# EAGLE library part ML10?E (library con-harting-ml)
HARTING
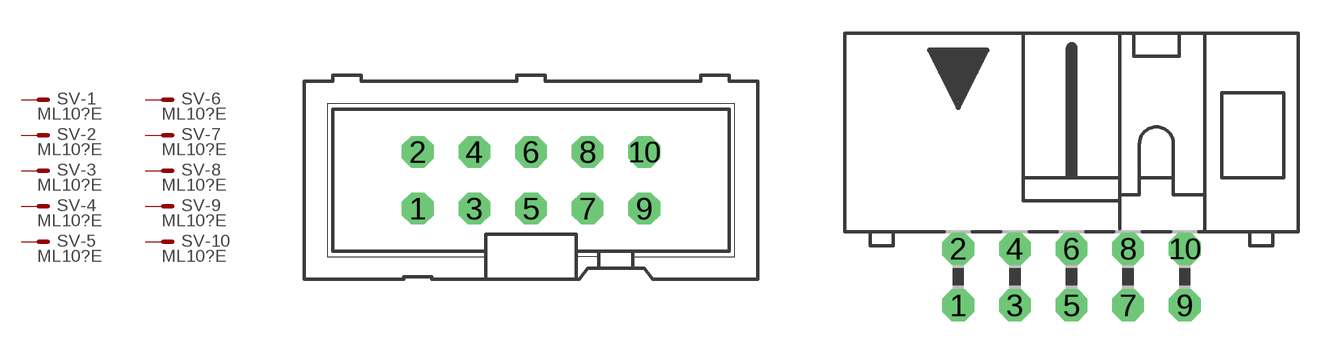
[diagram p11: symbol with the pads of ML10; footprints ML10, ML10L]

Designator prefix SV; gates -1=M -2=M -3=M -4=M -5=M -6=M -7=M -8=M -9=M -10=M

## ML10E (OC_FARNELL: unknown; OC_NEWARK: unknown)  [ML10]
1  -1:S  pas
2  -2:S  pas
3  -3:S  pas
4  -4:S  pas
5  -5:S  pas
6  -6:S  pas
7  -7:S  pas
8  -8:S  pas
9  -9:S  pas
10  -10:S  pas

## ML10LE (OC_FARNELL: unknown; OC_NEWARK: unknown)  [ML10L]
Pads as for ML10

## ML10-3ME (OC_FARNELL: unknown; OC_NEWARK: unknown)  [3M_10]
Pads as for ML10

## ML10-3MLE (OC_FARNELL: unknown; OC_NEWARK: unknown)  [3M_10L]
Pads as for ML10

## Footprint ML10 (pad centres in mm)
HARTING
drill 0.914 octagon: 1 -5.08,-1.27; 2 -5.08,1.27; 3 -2.54,-1.27; 4 -2.54,1.27; 5 0,-1.27; 6 0,1.27; 7 2.54,-1.27; 8 2.54,1.27; 9 5.08,-1.27; 10 5.08,1.27

## Footprint ML10L (pad centres in mm)
HARTING
drill 0.914 octagon: 1 -5.08,-1.27; 2 -5.08,1.27; 3 -2.54,-1.27; 4 -2.54,1.27; 5 0,-1.27; 6 0,1.27; 7 2.54,-1.27; 8 2.54,1.27; 9 5.08,-1.27; 10 5.08,1.27

## Footprint 3M_10 (pad centres in mm)
3M
drill 0.813 square: 1 -5.08,-1.27; 2 -5.08,1.27; 3 -2.54,-1.27; 4 -2.54,1.27; 5 0,-1.27; 6 0,1.27; 7 2.54,-1.27; 8 2.54,1.27; 9 5.08,-1.27; 10 5.08,1.27

## Footprint 3M_10L (pad centres in mm)
3M
drill 0.813 square: 1 -5.08,-5.08; 2 -5.08,-2.54; 3 -2.54,-5.08; 4 -2.54,-2.54; 5 0,-5.08; 6 0,-2.54; 7 2.54,-5.08; 8 2.54,-2.54; 9 5.08,-5.08; 10 5.08,-2.54
hole 2.54 at -10.998,-3.277
hole 2.54 at 10.998,-3.277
